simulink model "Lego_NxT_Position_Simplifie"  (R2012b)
settings: Solver=ode45  StartTime=0.0  StopTime=1  RelTol=1e-3

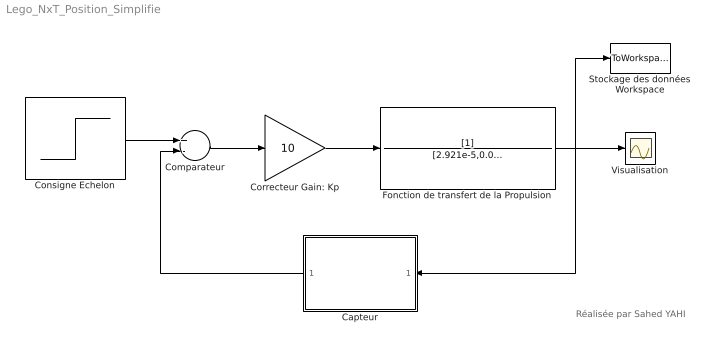
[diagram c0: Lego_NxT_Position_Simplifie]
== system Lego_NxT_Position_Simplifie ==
  note: Réalisée par Sahed YAHI
  Capteur : Subsystem
  Comparateur : Sum  Inputs=+-
  Consigne Echelon : Step  Time=0  After=90  SampleTime=0
  Correcteur Gain: Kp : Gain  Gain=10
  Fonction de transfert de la Propulsion : TransferFcn  Denominator=[2.921e-5,0.0315, 0.5048,0]
  Stockage des données Workspace : ToWorkspace  VariableName=simData  SampleTime=-1  SaveFormat=Timeseries
  Visualisation : Scope
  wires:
  Fonction de transfert de la Propulsion/1 -> Capteur/1(In1), Stockage des données Workspace/1, Visualisation/1
  Comparateur/1 -> Correcteur Gain: Kp/1
  Correcteur Gain: Kp/1 -> Fonction de transfert de la Propulsion/1
  Capteur/1(Out1) -> Comparateur/2
  Consigne Echelon/1 -> Comparateur/1

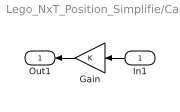
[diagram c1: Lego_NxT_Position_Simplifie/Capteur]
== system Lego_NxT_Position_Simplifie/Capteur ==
  In1 : Inport
  Gain : Gain
  Out1 : Outport
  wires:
  In1/1 -> Gain/1
  Gain/1 -> Out1/1
